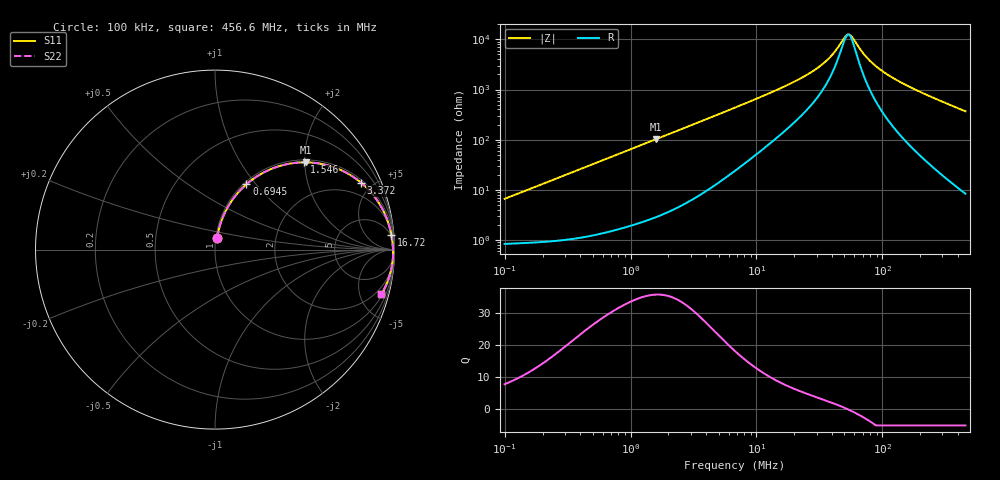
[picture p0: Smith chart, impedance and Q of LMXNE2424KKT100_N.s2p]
! LMXNE2424KKT100_N  S-PARAMETER MODEL  ( General Type )
! Model Generated by TAIYO YUDEN Corporation (http://www.ty-top.com)
! Version 1.0
! TAIYO YUDEN Control No. 191023NI43SB-FBB
! Copyright(c) 2019 TAIYO YUDEN CO.,LTD. All Rights Reserved.
! Product Description (link to TY-COMPAS)
! https://ds.yuden.co.jp/TYCOMPAS/or/detail?pn=LMXNE2424KKT100MN&u=M
! Products Name : Inductors
! Characteristics :
!  Inductance : 10 uH , SRF(min) : 32 MHz , DC Resistance(max) : 0.828 Ohm
!  Rated Current : Saturation :550 mA , Temp Rise : 450 mA
!  Case Size : 2.4 x 2.4 / 0.094 x 0.094 [mm/inch] , Thickness : 1 / 0.039 [mm/inch]
!  (Conditions: Temperature = 25 degC , DC Bias Current/Voltage = 0A / 0V)
! External Node Assignments :
!  1  o---GGG---o  2
! GND o---------o GND
! Frequency Range : 0.1MHz  -  456.598367MHz  [ 402 STEP ]
# MHz S RI R 50
! Freq[MHz].  S11 Real  S11 Imag  S21 Real  S21 Imag  S12 Real  S12 Imag  S22 Real  S22 Imag
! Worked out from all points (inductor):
!   401 points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, 100 kHz to 456.6 MHz, reference 50 ohm
!   read as one part in series: L = 10.4 uH near 104.3 kHz
!   highest Q = 35.9 at 1.579 MHz (marker M1), where L = 10.2 uH
!   self-resonance near 53.25 MHz
!   S11 on the Smith chart (normalised r, x): 100 kHz: 1.02, +0.13; 694.5 kHz: 1.03, +0.89; 1.546 MHz: 1.06, +1.98; 3.372 MHz: 1.14, +4.31; 16.72 MHz: 4, +23; 456.6 MHz: 1.17, -7.37
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0.1  0.0124 0.0641  0.9876 -0.0641  0.9876 -0.0641  0.0124 0.0641
0.20903  0.0267 0.131  0.9733 -0.131  0.9733 -0.131  0.0267 0.131
0.410178  0.0747 0.2428  0.9253 -0.2428  0.9253 -0.2428  0.0747 0.2428
0.694533  0.1749 0.3637  0.8251 -0.3637  0.8251 -0.3637  0.1749 0.3637
1.080982  0.3296 0.4557  0.6704 -0.4557  0.6704 -0.4557  0.3296 0.4557
1.546496  0.4951 0.4862  0.5049 -0.4862  0.5049 -0.4862  0.4951 0.4862
1.57942  0.5053 0.4862  0.4947 -0.4862  0.4947 -0.4862  0.5053 0.4862
1.682457  0.5358 0.485  0.4642 -0.485  0.4642 -0.485  0.5358 0.485
3.371752  0.8149 0.3719  0.1851 -0.3719  0.1851 -0.3719  0.8149 0.3719
6.901063  0.9415 0.2085  0.0585 -0.2085  0.0585 -0.2085  0.9415 0.2085
16.71734  0.982 0.0835  0.018 -0.0835  0.018 -0.0835  0.982 0.0835
27.71655  0.9884 0.0418  0.0116 -0.0418  0.0116 -0.0418  0.9884 0.0418
37.22399  0.9905 0.0224  0.0095 -0.0224  0.0095 -0.0224  0.9905 0.0224
42.23922  0.9912 0.0145  0.00882 -0.0145  0.00882 -0.0145  0.9912 0.0145
49.9927  0.9919 0.00422  0.00812 -0.00422  0.00812 -0.00422  0.9919 0.00422
54.38786  0.9921 -0.000936  0.00785 0.000936  0.00785 0.000936  0.9921 -0.000936
57.93599  0.9923 -0.00484  0.0077 0.00484  0.0077 0.00484  0.9923 -0.00484
68.57079  0.9925 -0.0155  0.00748 0.0155  0.00748 0.0155  0.9925 -0.0155
79.46593  0.9925 -0.0252  0.00755 0.0252  0.00755 0.0252  0.9925 -0.0252
113.6871  0.991 -0.0519  0.00904 0.0519  0.00904 0.0519  0.991 -0.0519
200.7843  0.9819 -0.1094  0.0181 0.1094  0.0181 0.1094  0.9819 -0.1094
456.5984  0.9265 -0.2499  0.0735 0.2499  0.0735 0.2499  0.9265 -0.2499
